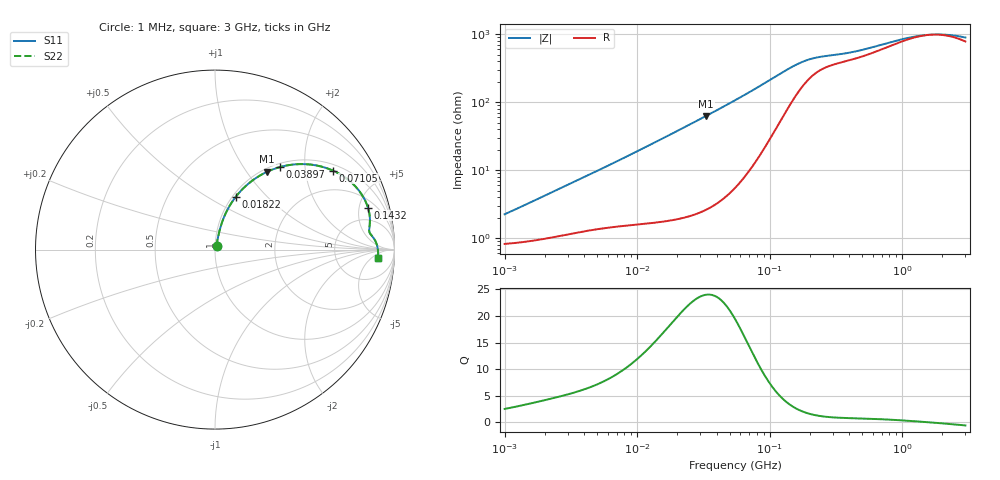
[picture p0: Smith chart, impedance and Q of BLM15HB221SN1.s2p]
! BLM15HB221SN1
# Hz S RI R 50
!Freq.(Hz) S11(Real) S11(Imag) S21(Real) S21(Imag) S12(Real) S12(Imag) S22(Real) S22(Imag)
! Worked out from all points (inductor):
!   401 points, 1 MHz to 3 GHz, reference 50 ohm
!   read as one part in series: L = 328 nH near 1.246 MHz
!   highest Q = 24 at 33.21 MHz (marker M1), where L = 300 nH
!   self-resonance near 1.667 GHz
!   S11 on the Smith chart (normalised r, x): 1 MHz: 1.02, +0.04; 18.22 MHz: 1.04, +0.68; 38.97 MHz: 1.06, +1.48; 71.05 MHz: 1.20, +2.82; 143.2 MHz: 2.85, +6.10; 3 GHz: 17, -9
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1000000  0.00855 0.0205  0.9914 -0.0205  0.9914 -0.0205  0.00855 0.0205
3823119  0.0176 0.0727  0.9824 -0.0727  0.9824 -0.0727  0.0176 0.0727
7858845  0.0355 0.1413  0.9645 -0.1413  0.9645 -0.1413  0.0355 0.1413
1.461624e7  0.0831 0.2464  0.9169 -0.2464  0.9169 -0.2464  0.0831 0.2464
1.821614e7  0.1167 0.2954  0.8833 -0.2954  0.8833 -0.2954  0.1167 0.2954
2.459509e7  0.1862 0.3673  0.8138 -0.3673  0.8138 -0.3673  0.1862 0.3673
3.320783e7  0.2899 0.4333  0.7101 -0.4333  0.7101 -0.4333  0.2899 0.4333
3.897472e7  0.3594 0.4592  0.6406 -0.4592  0.6406 -0.4592  0.3594 0.4592
5.477226e7  0.5283 0.4741  0.4717 -0.4741  0.4717 -0.4741  0.5283 0.4741
7.105049e7  0.6563 0.4405  0.3437 -0.4405  0.3437 -0.4405  0.6563 0.4405
8.507507e7  0.732 0.3968  0.268 -0.3968  0.268 -0.3968  0.732 0.3968
1.018679e8  0.791 0.3422  0.209 -0.3422  0.209 -0.3422  0.791 0.3422
1.431579e8  0.8521 0.2343  0.1479 -0.2343  0.1479 -0.2343  0.8521 0.2343
1.748812e8  0.8625 0.1815  0.1375 -0.1815  0.1375 -0.1815  0.8625 0.1815
2.094008e8  0.8627 0.1459  0.1373 -0.1459  0.1373 -0.1459  0.8627 0.1459
2.827291e8  0.8589 0.1102  0.1411 -0.1102  0.1411 -0.1102  0.8589 0.1102
4.570858e8  0.8689 0.0832  0.1311 -0.0832  0.1311 -0.0832  0.8689 0.0832
8.005644e8  0.8923 0.0503  0.1077 -0.0503  0.1077 -0.0503  0.8923 0.0503
1.171007e9  0.9026 0.0246  0.0974 -0.0246  0.0974 -0.0246  0.9026 0.0246
1.613037e9  0.9072 0.00231  0.0928 -0.00231  0.0928 -0.00231  0.9072 0.00231
2.177892e9  0.9089 -0.0195  0.0911 0.0195  0.0911 0.0195  0.9089 -0.0195
3e9  0.9083 -0.0451  0.0917 0.0451  0.0917 0.0451  0.9083 -0.0451
